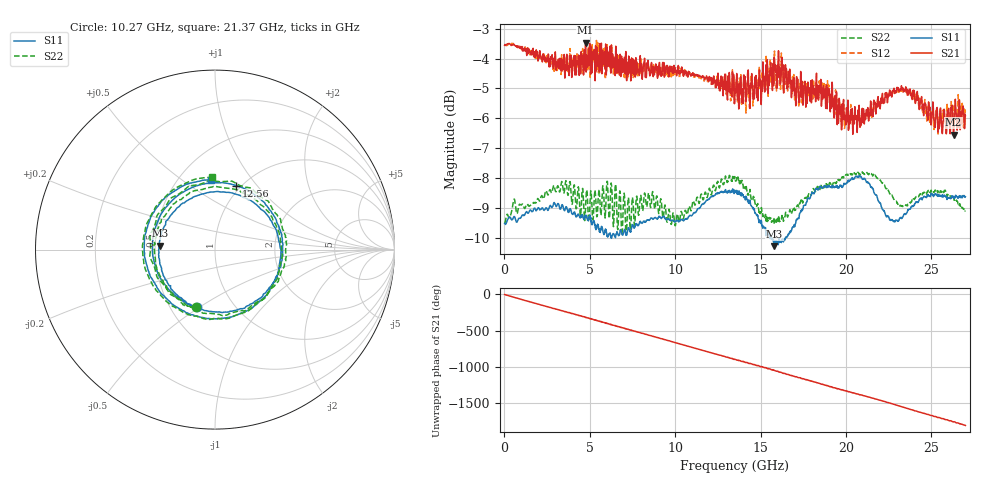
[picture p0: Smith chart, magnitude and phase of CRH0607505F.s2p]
!Agilent Technologies,N5224A,MY51441447,A.10.00.00
!Agilent N5224A: A.10.00.00
!Date: Thursday, November 05, 2015 12:21:42
!Correction: S11(Full 2 Port(1,2))
!S21(Full 2 Port(1,2))
!S12(Full 2 Port(1,2))
!S22(Full 2 Port(1,2))
!S2P File: Measurements: S11, S21, S12, S22:
# Hz S  RI  R 50
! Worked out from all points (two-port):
!   1601 points, 10 MHz to 27 GHz, reference 50 ohm
!   highest |S21| = -3.47 dB at 4.75 GHz (marker M1); lowest = -6.5 dB at 26.31 GHz (marker M2)
!   |S21| within 3 dB of the highest: start of sweep to 20.4 GHz; 20.66 GHz to 25.64 GHz (4.986 GHz wide, 21.5 % of centre)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
!   lowest |S11| = -10.3 dB at 15.8 GHz (marker M3), VSWR 1.88, Z = 26.6 + j1.24 ohm
!   |S11| at or under -10 dB: 6.261955 GHz to 6.275201 GHz (13.25 MHz wide, 0.211 % of centre); 15.54184 GHz to 15.58186 GHz (40.02 MHz wide, 0.257 % of centre); 15.61 GHz to 16.46 GHz (848.6 MHz wide, 5.29 % of centre)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
!   |S22| runs from -9.9 to -7.8 dB; largest |S21 - S12| = 0.074
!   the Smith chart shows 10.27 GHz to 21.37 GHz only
!   S11 on the Smith chart (normalised r, x): 10.27 GHz: 0.68, -0.49; 12.56 GHz: 0.95, +0.79; 21.37 GHz: 0.71, +0.65
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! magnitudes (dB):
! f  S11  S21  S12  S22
! 10 MHz  -9.5  -3.6  -3.5  -9.5
! 3.266 GHz  -9.0  -4.3  -4.2  -8.4
! 4.514 GHz  -9.3  -4.0  -3.8  -8.8
! 4.75 GHz  -9.2  -3.5  -4.0  -9.0
! 6.37 GHz  -9.9  -4.3  -4.2  -9.5
! 7.247 GHz  -9.7  -4.4  -4.3  -8.7
! 9.018 GHz  -9.3  -4.4  -4.6  -9.1
! 10.27 GHz  -9.4  -4.4  -4.6  -9.4
! 12.56 GHz  -8.5  -5.0  -4.8  -8.3
! 13.51 GHz  -8.5  -5.0  -5.0  -8.0
! 14.25 GHz  -8.8  -4.8  -4.4  -8.6
! 15.8 GHz  -10.3  -4.0  -4.1  -9.5
! 16.47 GHz  -10.0  -4.5  -4.3  -9.1
! 18.01 GHz  -8.5  -5.0  -5.1  -8.5
! 18.87 GHz  -8.3  -4.9  -5.4  -8.2
! 20.05 GHz  -8.2  -5.7  -5.8  -7.9
! 21.37 GHz  -8.2  -5.8  -5.9  -7.8
! 22.51 GHz  -9.3  -5.3  -5.2  -8.5
! 23.83 GHz  -9.0  -5.2  -5.2  -8.8
! 25.28 GHz  -8.6  -5.9  -5.7  -8.4
! 26.31 GHz  -8.6  -6.5  -6.0  -8.6
! 27 GHz  -8.6  -5.9  -5.8  -9.1
